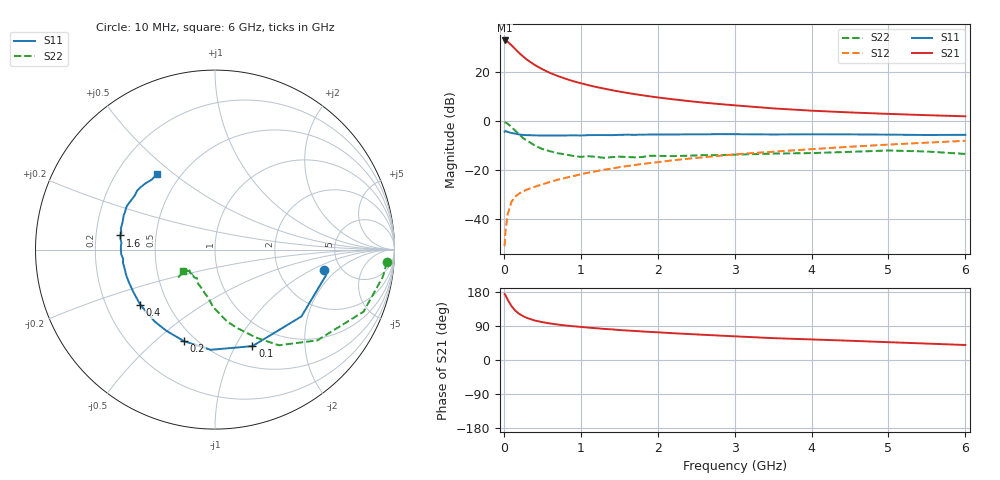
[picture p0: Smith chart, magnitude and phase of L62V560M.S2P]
!  INFINEON TECHNOLOGIES Small Signal Semiconductors
! BFR380L3 , Si-NPN RF-Transistor in TSLP-3-1
!  Vce=2.5 V,  Ic=60 mA
! Common Emitter S-Parameters:  07. March 2005
#  GHz  S  MA  R  50
! f  S11  S21  S12  S22
! GHz  Mag  Ang  Mag  Ang  Mag  Ang  Mag  Ang
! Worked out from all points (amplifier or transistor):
!   36 points, 10 MHz to 6 GHz, reference 50 ohm
!   highest |S21| = 33.1 dB at 10 MHz (marker M1)
!   |S21| within 3 dB of that: start of sweep to 132.3 MHz
!   unconditionally stable (mu >= 1): 1.359 GHz to 4.856 GHz
!   at 250 MHz: K = 0.52, MSG = 27.6 dB, |S12| = -28.7 dB
!   at 1.4 GHz: K = 1.00, MAG = 15.6 dB, |S12| = -19.3 dB
!   at 6 GHz: K = 0.98, MSG = 5.0 dB, |S12| = -8.0 dB
!   S11 on the Smith chart (normalised r, x): 10 MHz: 3.69, -1.32; 100 MHz: 0.73, -1.17; 200 MHz: 0.43, -0.63; 400 MHz: 0.35, -0.29; 1.6 GHz: 0.31, +0.07; 6 GHz: 0.37, +0.44
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0.01  0.6152 -10.4  45.14 174.0  0.0028 79.0  0.96 -4.2
0.02  0.6345 -13.1  44.57 171.6  0.0055 85.2  0.9469 -9.3
0.05  0.6087 -37.7  42.32 158.9  0.0126 74.9  0.8967 -22.7
0.1  0.5768 -68.8  36.01 142.2  0.0228 63.0  0.762 -41.6
0.15  0.5588 -92.5  29.93 130.0  0.029 57.7  0.6414 -56.2
0.2  0.539 -108.5  24.97 121.7  0.0335 55.6  0.5396 -65.1
0.25  0.5274 -120.9  21.26 115.7  0.0368 53.4  0.4555 -74.0
0.3  0.5229 -130.0  18.29 111.0  0.0402 53.8  0.4066 -80.4
0.4  0.5174 -143.6  14.29 104.3  0.0458 54.8  0.322 -91.6
0.5  0.5126 -152.6  11.67 99.9  0.0515 57.1  0.2721 -97.8
0.6  0.5131 -158.9  9.786 96.4  0.0577 58.4  0.2448 -104.4
0.7  0.5148 -163.5  8.476 93.6  0.0641 60.9  0.2229 -111.0
0.9  0.5181 -172.0  6.638 89.1  0.0759 63.0  0.1965 -121.3
1.1  0.5227 -177.0  5.493 85.4  0.0893 64.6  0.1934 -126.5
1.3  0.5246 177.6  4.686 82.1  0.1025 65.7  0.1793 -133.9
1.6  0.5334 171.5  3.826 77.8  0.1216 66.3  0.1867 -140.6
2.2  0.5377 162.8  2.823 70.7  0.1599 66.7  0.1946 -141.9
2.8  0.5476 154.4  2.26 64.5  0.1974 66.3  0.2039 -147.2
3.5  0.5393 146.2  1.842 57.7  0.2395 64.1  0.2193 -145.3
4.5  0.5413 140.2  1.522 50.8  0.3024 62.1  0.2377 -144.1
5.5  0.5257 132.2  1.337 43.3  0.3667 58.1  0.2417 -143.6
6  0.5306 127.2  1.268 39.6  0.3996 55.8  0.2155 -146.2
